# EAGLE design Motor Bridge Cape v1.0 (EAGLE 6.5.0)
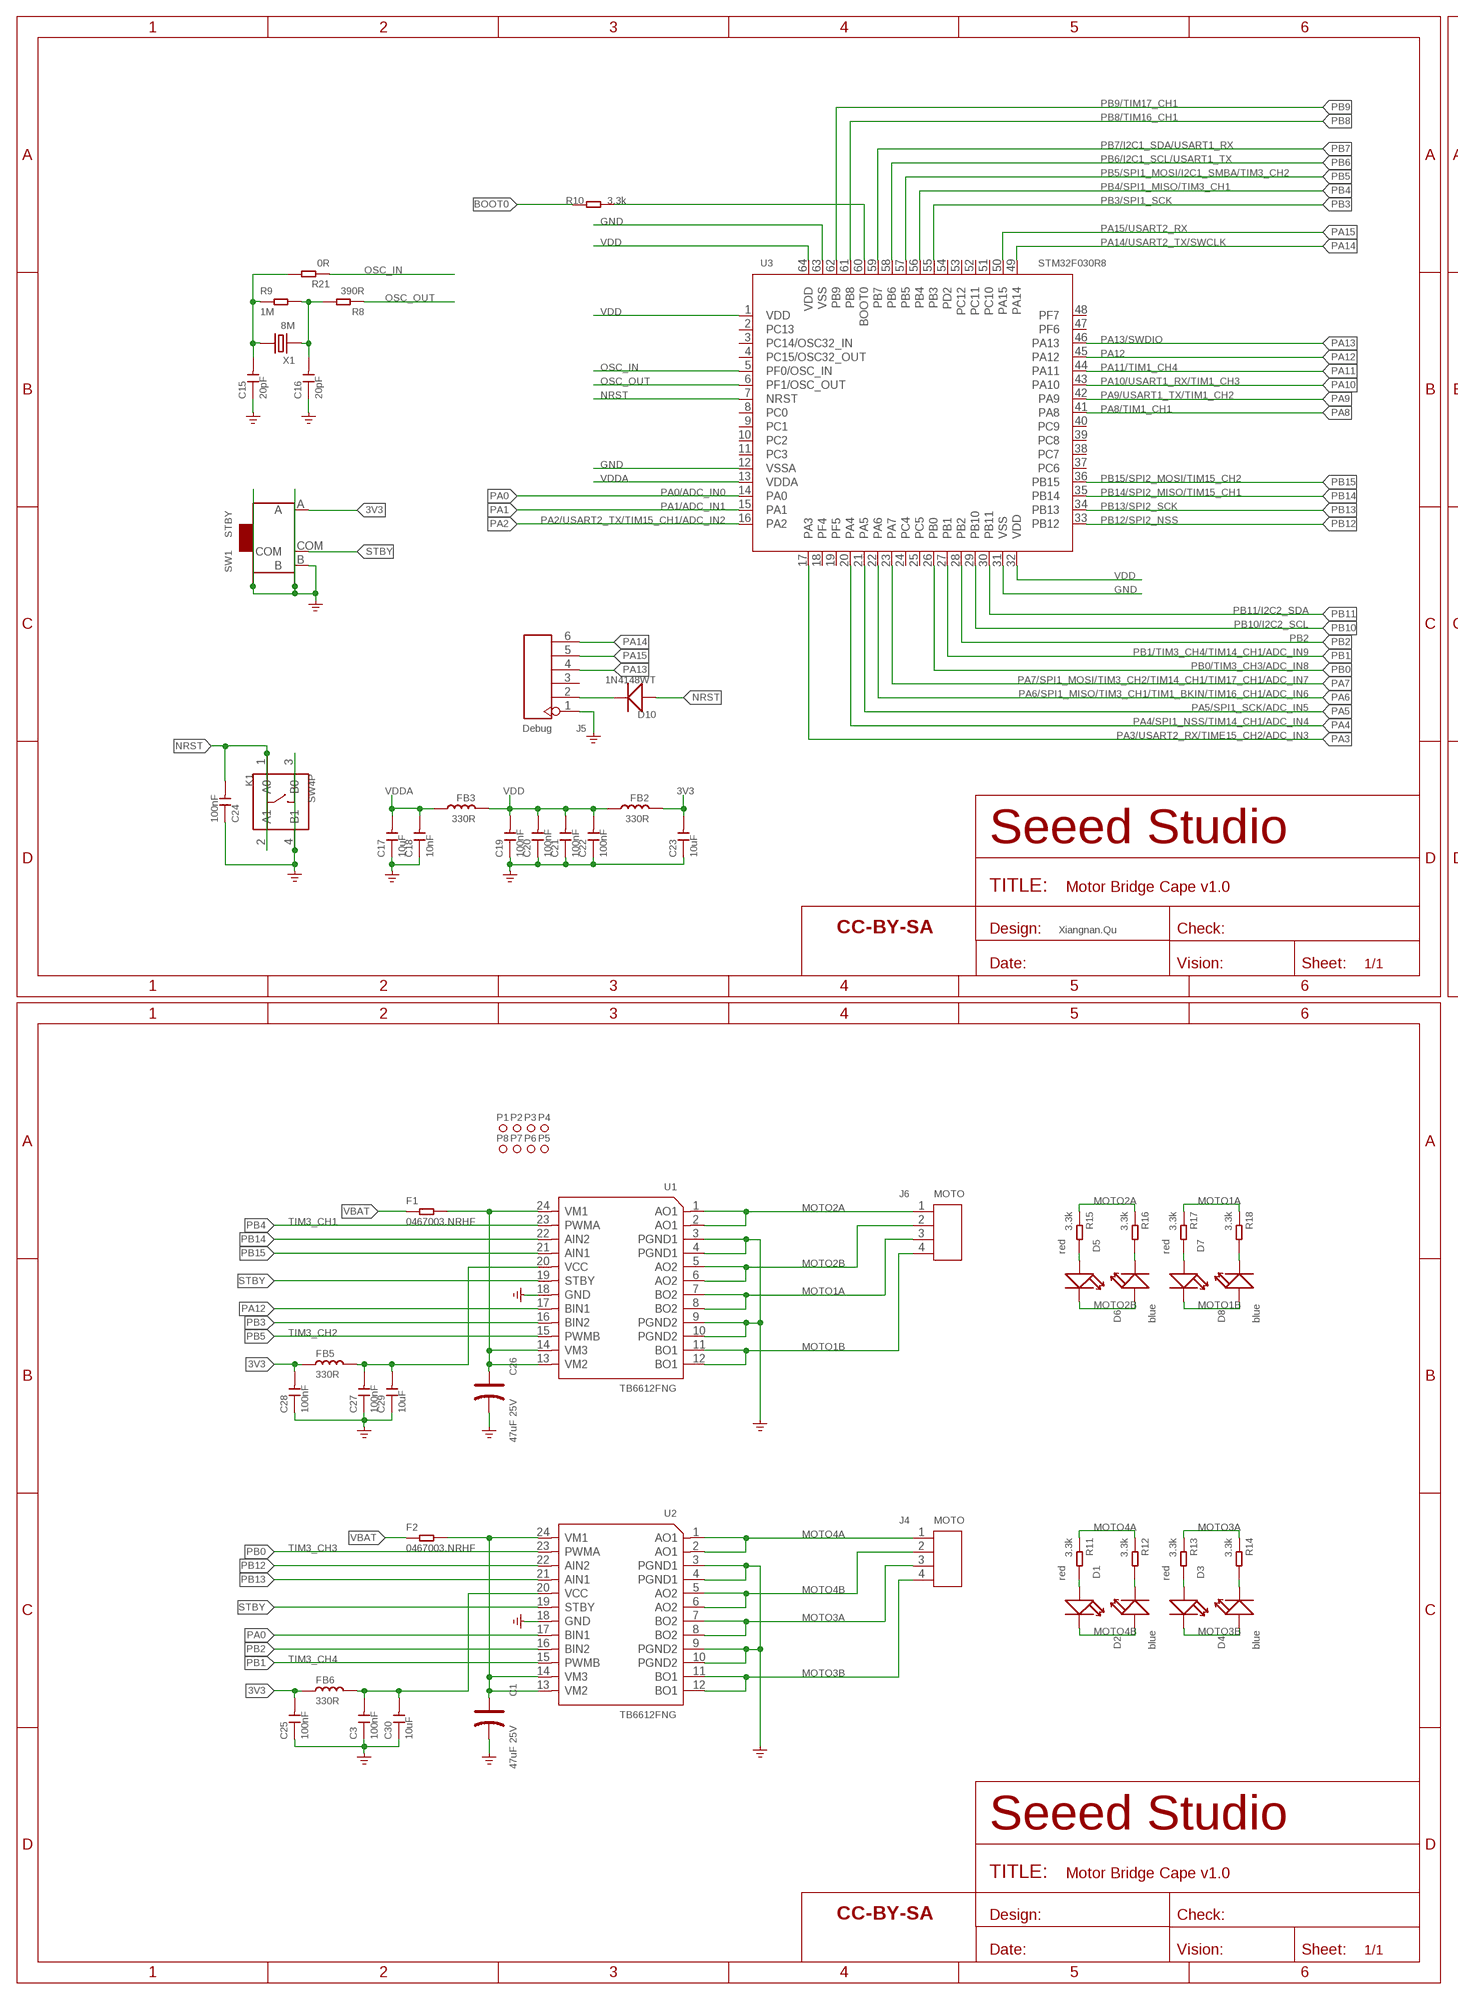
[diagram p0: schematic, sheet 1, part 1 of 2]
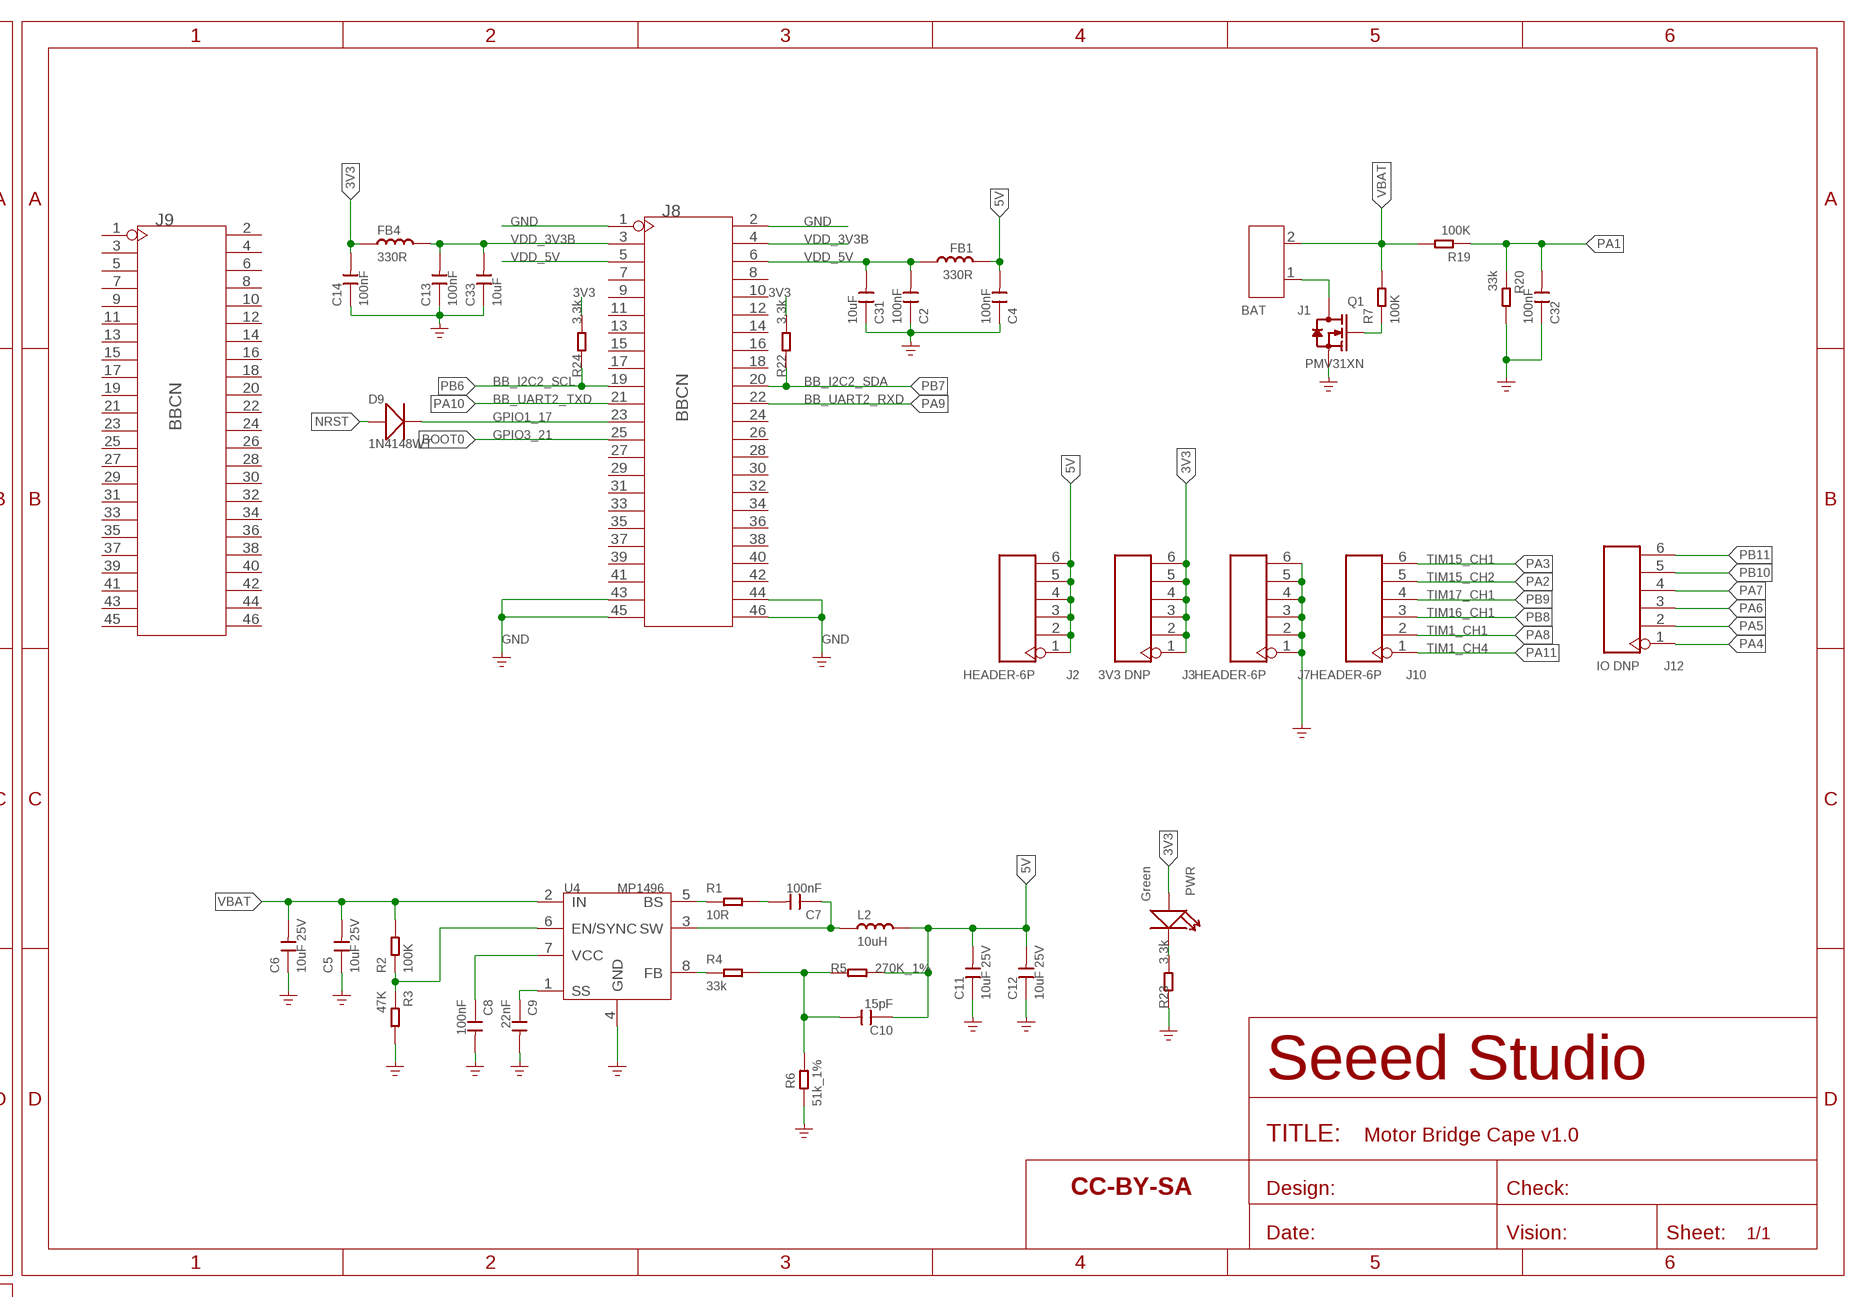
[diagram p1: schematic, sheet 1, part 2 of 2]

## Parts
C1  47uF 25V  CAP-POLAR-ELECTRO-C  [ELECTRO-SMD-C-6MM]
C2  100nF  CAP-0603  [C0603]
C3  100nF  CAP-0603  [C0603]
C4  100nF  CAP-0603  [C0603]
C5  10uF 25V  CAP-0805  [C0805]
C6  10uF 25V  CAP-0805  [C0805]
C7  100nF  CAP-0603  [C0603]
C8  100nF  CAP-0603  [C0603]
C9  22nF  CAP-0603  [C0603]
C10  15pF  CAP-0603  [C0603]
C11  10uF 25V  CAP-0805  [C0805]
C12  10uF 25V  CAP-0805  [C0805]
C13  100nF  CAP-0603  [C0603]
C14  100nF  CAP-0603  [C0603]
C15  20pF  CAP-0603  [C0603]
C16  20pF  CAP-0603  [C0603]
C17  10uF  CAP-0603  [C0603]
C18  10nF  CAP-0603  [C0603]
C19  100nF  CAP-0603  [C0603]
C20  100nF  CAP-0603  [C0603]
C21  100nF  CAP-0603  [C0603]
C22  100nF  CAP-0603  [C0603]
C23  10uF  CAP-0603  [C0603]
C24  100nF  CAP-0603  [C0603]
C25  100nF  CAP-0603  [C0603]
C26  47uF 25V  CAP-POLAR-ELECTRO-C  [ELECTRO-SMD-C-6MM]
C27  100nF  CAP-0603  [C0603]
C28  100nF  CAP-0603  [C0603]
C29  10uF  CAP-0603  [C0603]
C30  10uF  CAP-0603  [C0603]
C31  10uF  CAP-0603  [C0603]
C32  100nF  CAP-0603  [C0603]
C33  10uF  CAP-0603  [C0603]
D1  red  LED'0603'  [LED-0603]
D2  blue  LED'0603'  [LED-0603]
D3  red  LED'0603'  [LED-0603]
D4  blue  LED'0603'  [LED-0603]
D5  red  LED'0603'  [LED-0603]
D6  blue  LED'0603'  [LED-0603]
D7  red  LED'0603'  [LED-0603]
D8  blue  LED'0603'  [LED-0603]
D9  1N4148WT  DIODE'0603'  [SOD-523]
D10  1N4148WT  DIODE'0603'  [SOD-523]
F1  0467003.NRHF  RES-0603  [R0603]
F2  0467003.NRHF  RES-0603  [R0603]
FB1  330R  INDUCTOR/FERRITE-BEAD'0603'  [L0603]
FB2  330R  INDUCTOR/FERRITE-BEAD'0603'  [L0603]
FB3  330R  INDUCTOR/FERRITE-BEAD'0603'  [L0603]
FB4  330R  INDUCTOR/FERRITE-BEAD'0603'  [L0603]
FB5  330R  INDUCTOR/FERRITE-BEAD'0603'  [L0603]
FB6  330R  INDUCTOR/FERRITE-BEAD'0603'  [L0603]
FR1  SEEEDSTUDIO-OPEN-SCH-FRAME  [SEEEDSTUDIO-PCB-FRAME]
FR2  SEEEDSTUDIO-OPEN-SCH-FRAME  [SEEEDSTUDIO-PCB-FRAME]
FR4  SEEEDSTUDIO-OPEN-SCH-FRAME  [SEEEDSTUDIO-PCB-FRAME]
J1  BAT  SCREW-TERMINAL-2P'3.5'  [H2-3.5-7.0X7.0MM]
J2  HEADER-6P  HEADER-6P-65/35MIL  [H6-2.54-C65D35MIL]
J3  3V3 DNP  HEADER-6P-65/35MIL  [H6-2.54-C65D35MIL]
J4  MOTO  SCREW-TERMINAL-4P'3.5'  [H4-3.5-14.0X7.0MM]
J5  Debug  HEADER-6P-65/35MIL  [H6-2.54-C65D35MIL]
J6  MOTO  SCREW-TERMINAL-4P'3.5'  [H4-3.5-14.0X7.0MM]
J7  HEADER-6P  HEADER-6P-65/35MIL  [H6-2.54-C65D35MIL]
J8  BBCN  HEADER-2X23P  [2X23P-2.54]
J9  BBCN  HEADER-2X23P  [2X23P-2.54]
J10  HEADER-6P  HEADER-6P-65/35MIL  [H6-2.54-C65D35MIL]
J12  IO DNP  HEADER-6P-65/35MIL  [H6-2.54-C65D35MIL]
K1  SW4P  BUTTON-4P  [SW4P-SMD-4.5X3.2X2.5MM]
L2  10uH  INDUCTOR/FERRITE-BEAD'1813'  [L1813]
P1  MARK-1.0'ANNULAR'  [ROUND-MARK-1.0]
P2  MARK-1.0'ANNULAR'  [ROUND-MARK-1.0]
P3  MARK-1.0'ANNULAR'  [ROUND-MARK-1.0]
P4  MARK-1.0'ANNULAR'  [ROUND-MARK-1.0]
P5  MARK-1.0'ANNULAR'  [ROUND-MARK-1.0]
P6  MARK-1.0'ANNULAR'  [ROUND-MARK-1.0]
P7  MARK-1.0'ANNULAR'  [ROUND-MARK-1.0]
P8  MARK-1.0'ANNULAR'  [ROUND-MARK-1.0]
PWR  Green  LED'0603'  [LED-0603]
Q1  PMV31XN  MOSFET-N'SOT23'  [SOT-23]
R1  10R  RES-0603  [R0603]
R2  100K  RES-0603  [R0603]
R3  47K  RES-0603  [R0603]
R4  33k  RES-0603  [R0603]
R5  270K_1%  RES-0603  [R0603]
R6  51k_1%  RES-0603  [R0603]
R7  100K  RES-0603  [R0603]
R8  390R  RES-0603  [R0603]
R9  1M  RES-0603  [R0603]
R10  3.3k  RES-0603  [R0603]
R11  3.3k  RES-0603  [R0603]
R12  3.3k  RES-0603  [R0603]
R13  3.3k  RES-0603  [R0603]
R14  3.3k  RES-0603  [R0603]
R15  3.3k  RES-0603  [R0603]
R16  3.3k  RES-0603  [R0603]
R17  3.3k  RES-0603  [R0603]
R18  3.3k  RES-0603  [R0603]
R19  100K  RES-0603  [R0603]
R20  33k  RES-0603  [R0603]
R21  0R  RES-0603  [R0603]
R22  3.3k  RES-0603  [R0603]
R23  3.3k  RES-0603  [R0603]
R24  3.3k  RES-0603  [R0603]
SW1  STBY  SWITCH-3+4P  [SW7-SMD-L6.7X2.7X3.2MM]
U1  TB6612FNG  DRIVER-TB6612FNG  [SSOP24-0.65-8.3X5.6MM]
U2  TB6612FNG  DRIVER-TB6612FNG  [SSOP24-0.65-8.3X5.6MM]
U3  STM32F030R8  MCU-STM32F030R8  [LQFP64-0.5-10X10MM]
U4  MP1496  CONVERTER-MP1496DJ  [SOT-23-8]
X1  8M  CRYSTAL-2P'5032'  [X2-SMD-5.0X3.2X1.3MM]

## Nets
3V3: C14.2 C23.2 C25.2 C28.2 FB2.1 FB4.1 FB5.1 FB6.1 J3.1 J3.2 J3.3 J3.4 J3.5 J3.6 PWR.+ R22.1 R24.1 SW1.A
5V: C4.2 C10.1 C11.2 C12.2 FB1.1 J2.1 J2.2 J2.3 J2.4 J2.5 J2.6 L2.2 R5.2
BOOT0: J8.25 R10.2
GND: C1.- C2.1 C3.1 C4.1 C5.1 C6.1 C8.2 C9.2 C11.1 C12.1 C13.1 C14.1 C15.1 C16.1 C17.1 C18.1 C19.1 C20.1 C21.1 C22.1 C23.1 C24.1 C25.1 C26.- C27.1 C28.1 C29.1 C30.1 C31.1 C32.1 C33.1 J5.1 J7.1 J7.2 J7.3 J7.4 J7.5 J7.6 J8.1 J8.2 J8.43 J8.44 J8.45 J8.46 K1.3(B0) K1.4(B1) Q1.2(S) R3.2 R6.1 R20.2 R23.1 SW1.B SW1.SS1 SW1.SS2 SW1.SS3 SW1.SS4 U1.3(PGND1) U1.4(PGND1) U1.9(PGND2) U1.10(PGND2) U1.18(GND) U2.3(PGND1) U2.4(PGND1) U2.9(PGND2) U2.10(PGND2) U2.18(GND) U3.12(VSSA) U3.31(VSS) U3.63(VSS) U4.4(GND) ; supply symbol labelled GND_POWER
MOTO1A: J6.3 R17.1 R18.1 U1.7(BO2) U1.8(BO2)
MOTO1B: D7.- D8.+ J6.4 U1.11(BO1) U1.12(BO1)
MOTO2A: J6.1 R15.1 R16.1 U1.1(AO1) U1.2(AO1)
MOTO2B: D5.- D6.+ J6.2 U1.5(AO2) U1.6(AO2)
MOTO3A: J4.3 R13.1 R14.1 U2.7(BO2) U2.8(BO2)
MOTO3B: D3.- D4.+ J4.4 U2.11(BO1) U2.12(BO1)
MOTO4A: J4.1 R11.1 R12.1 U2.1(AO1) U2.2(AO1)
MOTO4B: D1.- D2.+ J4.2 U2.5(AO2) U2.6(AO2)
N$1: C10.2 R4.2 R5.1 R6.2
N$2: D3.+ R13.2
N$3: D4.- R14.2
N$4: C3.2 C30.2 FB6.2 U2.20(VCC)
N$5: R1.1 U4.5(BS)
N$6: C7.2 R1.2
N$7: C7.1 L2.1 U4.3(SW)
N$8: J1.1 Q1.3(D)
N$9: R4.1 U4.8(FB)
N$10: Q1.1(G) R7.1
N$11: D5.+ R15.2
N$12: C9.1 U4.1(SS)
N$13: C8.1 U4.7(VCC)
N$16: R2.1 R3.1 U4.6(EN/SYNC)
N$19: D1.+ R11.2
N$23: D2.- R12.2
N$24: D10.- J5.2
N$25: C16.2 R8.2 R9.2 X1.1
N$26: D6.- R16.2
N$27: C15.2 R9.1 R21.2 X1.2
N$28: R10.1 U3.60(BOOT0)
N$29: D7.+ R17.2
N$30: D8.- R18.2
N$31: C27.2 C29.2 FB5.2 U1.20(VCC)
N$32: C26.+ F1.2 U1.13(VM2) U1.14(VM3) U1.24(VM1)
N$34: C1.+ F2.2 U2.13(VM2) U2.14(VM3) U2.24(VM1)
N$44: PWR.- R23.2
N$60: D9.- J8.23
NRST: C24.2 D9.+ D10.+ K1.1(A0) K1.2(A1) U3.7(NRST)
OSC_IN: R21.1 U3.5(PF0/OSC_IN)
OSC_OUT: R8.1 U3.6(PF1/OSC_OUT)
PA0: U2.17(BIN1) U3.14(PA0)
PA1: C32.2 R19.1 R20.1 U3.15(PA1)
PA2: J10.5 U3.16(PA2)
PA3: J10.6 U3.17(PA3)
PA4: J12.1 U3.20(PA4)
PA5: J12.2 U3.21(PA5)
PA6: J12.3 U3.22(PA6)
PA7: J12.4 U3.23(PA7)
PA8: J10.2 U3.41(PA8)
PA9: J8.22 U3.42(PA9)
PA10: J8.21 U3.43(PA10)
PA11: J10.1 U3.44(PA11)
PA12: U1.17(BIN1) U3.45(PA12)
PA13: J5.4 U3.46(PA13)
PA14: J5.6 U3.49(PA14)
PA15: J5.5 U3.50(PA15)
PB0: U2.23(PWMA) U3.26(PB0)
PB1: U2.15(PWMB) U3.27(PB1)
PB2: U2.16(BIN2) U3.28(PB2)
PB3: U1.16(BIN2) U3.55(PB3)
PB4: U1.23(PWMA) U3.56(PB4)
PB5: U1.15(PWMB) U3.57(PB5)
PB6: J8.19 R24.2 U3.58(PB6)
PB7: J8.20 R22.2 U3.59(PB7)
PB8: J10.3 U3.61(PB8)
PB9: J10.4 U3.62(PB9)
PB10: J12.5 U3.29(PB10)
PB11: J12.6 U3.30(PB11)
PB12: U2.22(AIN2) U3.33(PB12)
PB13: U2.21(AIN1) U3.34(PB13)
PB14: U1.22(AIN2) U3.35(PB14)
PB15: U1.21(AIN1) U3.36(PB15)
STBY: SW1.COM U1.19(STBY) U2.19(STBY)
VBAT: C5.2 C6.2 F1.1 F2.1 J1.2 R2.2 R7.2 R19.2 U4.2(IN)
VDD: C19.2 C20.2 C21.2 C22.2 FB2.2 FB3.1 U3.1(VDD) U3.32(VDD) U3.64(VDD)
VDD_3V3B: C13.2 C33.2 FB4.2 J8.3 J8.4
VDD_5V: C2.2 C31.2 FB1.2 J8.5 J8.6
VDDA: C17.2 C18.2 FB3.2 U3.13(VDDA)
Unconnected: J5.3 J8.7 J8.8 J8.9 J8.10 J8.11 J8.12 J8.13 J8.14 J8.15 J8.16 J8.17 J8.18 J8.24 J8.26 J8.27 J8.28 J8.29 J8.30 J8.31 J8.32 J8.33 J8.34 J8.35 J8.36 J8.37 J8.38 J8.39 J8.40 J8.41 J8.42 J9.1 J9.2 J9.3 J9.4 J9.5 J9.6 J9.7 J9.8 J9.9 J9.10 J9.11 J9.12 J9.13 J9.14 J9.15 J9.16 J9.17 J9.18 J9.19 J9.20 J9.21 J9.22 J9.23 J9.24 J9.25 J9.26 J9.27 J9.28 J9.29 J9.30 J9.31 J9.32 J9.33 J9.34 J9.35 J9.36 J9.37 J9.38 J9.39 J9.40 J9.41 J9.42 J9.43 J9.44 J9.45 J9.46 U3.2(PC13) U3.3(PC14/OSC32_IN) U3.4(PC15/OSC32_OUT) U3.8(PC0) U3.9(PC1) U3.10(PC2) U3.11(PC3) U3.18(PF4) U3.19(PF5) U3.24(PC4) U3.25(PC5) U3.37(PC6) U3.38(PC7) U3.39(PC8) U3.40(PC9) U3.47(PF6) U3.48(PF7) U3.51(PC10) U3.52(PC11) U3.53(PC12) U3.54(PD2)

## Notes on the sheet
- PB9/TIM17_CH1
- PB8/TIM16_CH1
- PB7/I2C1_SDA/USART1_RX
- PB6/I2C1_SCL/USART1_TX
- PB5/SPI1_MOSI/I2C1_SMBA/TIM3_CH2
- PB4/SPI1_MISO/TIM3_CH1
- PB3/SPI1_SCK
- PA15/USART2_RX
- PA14/USART2_TX/SWCLK
- BB_I2C2_SCL | BB_I2C2_SDA
- BB_UART2_TXD | BB_UART2_RXD
- GPIO1_17
- PA13/SWDIO | GPIO3_21
- PA12
- PA11/TIM1_CH4
- PA10/USART1_RX/TIM1_CH3
- PA9/USART1_TX/TIM1_CH2
- PA8/TIM1_CH1
- TIM15_CH1
- TIM15_CH2
- TIM17_CH1
- PB15/SPI2_MOSI/TIM15_CH2 | TIM16_CH1
- PA0/ADC_IN0 | PB14/SPI2_MISO/TIM15_CH1 | TIM1_CH1
- PA1/ADC_IN1 | PB13/SPI2_SCK | TIM1_CH4
- PA2/USART2_TX/TIM15_CH1/ADC_IN2 | PB12/SPI2_NSS
- PB11/I2C2_SDA
- PB10/I2C2_SCL
- PB2
- PB1/TIM3_CH4/TIM14_CH1/ADC_IN9
- PB0/TIM3_CH3/ADC_IN8
- PA7/SPI1_MOSI/TIM3_CH2/TIM14_CH1/TIM17_CH1/ADC_IN7
- PA6/SPI1_MISO/TIM3_CH1/TIM1_BKIN/TIM16_CH1/ADC_IN6
- PA5/SPI1_SCK/ADC_IN5
- PA4/SPI1_NSS/TIM14_CH1/ADC_IN4
- PA3/USART2_RX/TIME15_CH2/ADC_IN3
- Xiangnan.Qu
- TIM3_CH1
- TIM3_CH2
- TIM3_CH3
- TIM3_CH4

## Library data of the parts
C1 C26 = Discrete-new:CAP-POLAR: Electrolytic Capacitors,Tantalum Capacitors and Super Capacitors
C2-C25 C27-C33 = Discrete-new:CAP: Ceramic Capacitors
D1-D8 PWR = Discrete-new:LED
D9 D10 = Discrete-new:DIODE*
F1 F2 R1-R24 = Discrete-new:RES
FB1-FB6 L2 = Discrete-new:INDUCTOR/FERRITE-BEAD
FR1 FR2 FR4 = moudle-new:SEEEDSTUDIO-OPEN-SCH-FRAME
J1 = Connector-new:SCREW-TERMINAL-2P: 2P-3.5:320110028;2P-5.0:320110031
J2 J3 J5 J7 J10 J12 = Connector-new:HEADER-6P
J4 J6 = Connector-new:SCREW-TERMINAL-4P: 203000033
J8 J9 = Connector :HEADER-2X23P
K1 = Discrete-new:BUTTON-4P: SW4-6.0X6.0X5.0MM:311020024;SW4-8.0X8.0X9.0MM:311020028;SW4-SMD-6.0X6.0X5.0MM:311020004;SW4-SMD-3.35X3.35X1.5MM:311020030;SW4-SMD-5.2X5.2X2.5MM:311020046
P1-P8 = Discrete-new:MARK-1.0; PARTNO: DNP
Q1 = Discrete-new:MOSFET-N
SW1 = Discrete-new:SWITCH-3+4P: SW7-SMD-6.7X2.6X1.4MM-90D:311030002;SW7-SMD-L6.7X2.7X3.2MM:311030001
U1 U2 = template:DRIVER-TB6612FNG; MPN: TB6612FNG
U3 = IC-new:MCU-STM32F030R8
U4 = template:CONVERTER-MP1496DJ: High-Efficiency,2A，16V,500kHz Synchronous,Step-Down Converter http://html.alldatasheetcn.com/html-pdf/551584/MPS/MP1496DJ/55/1/MP1496DJ.html
X1 = Discrete-new:CRYSTAL-2P

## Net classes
0 default: width 0.152 mm, drill 0.305 mm, clearance 0.152 mm

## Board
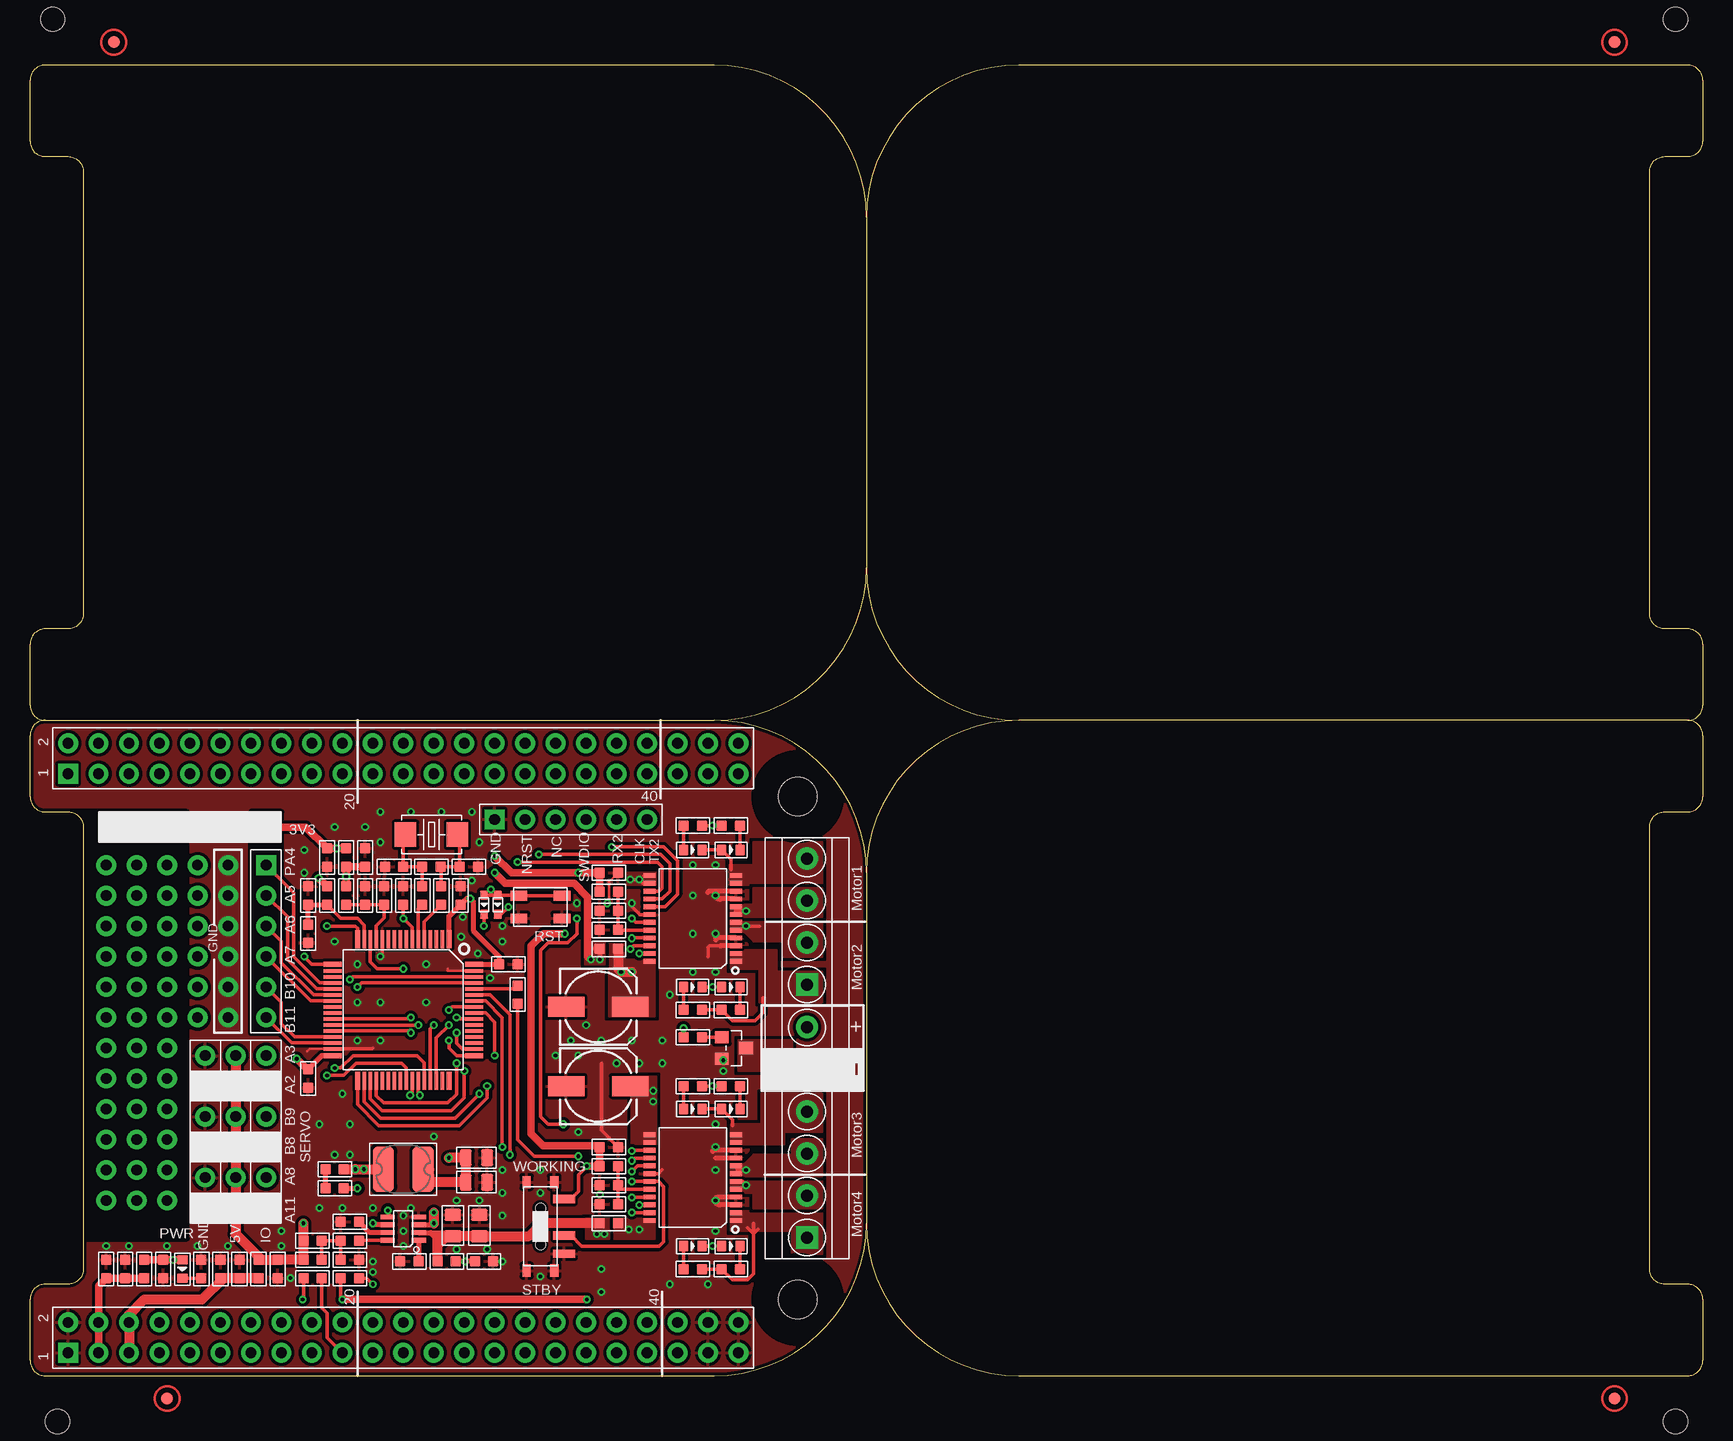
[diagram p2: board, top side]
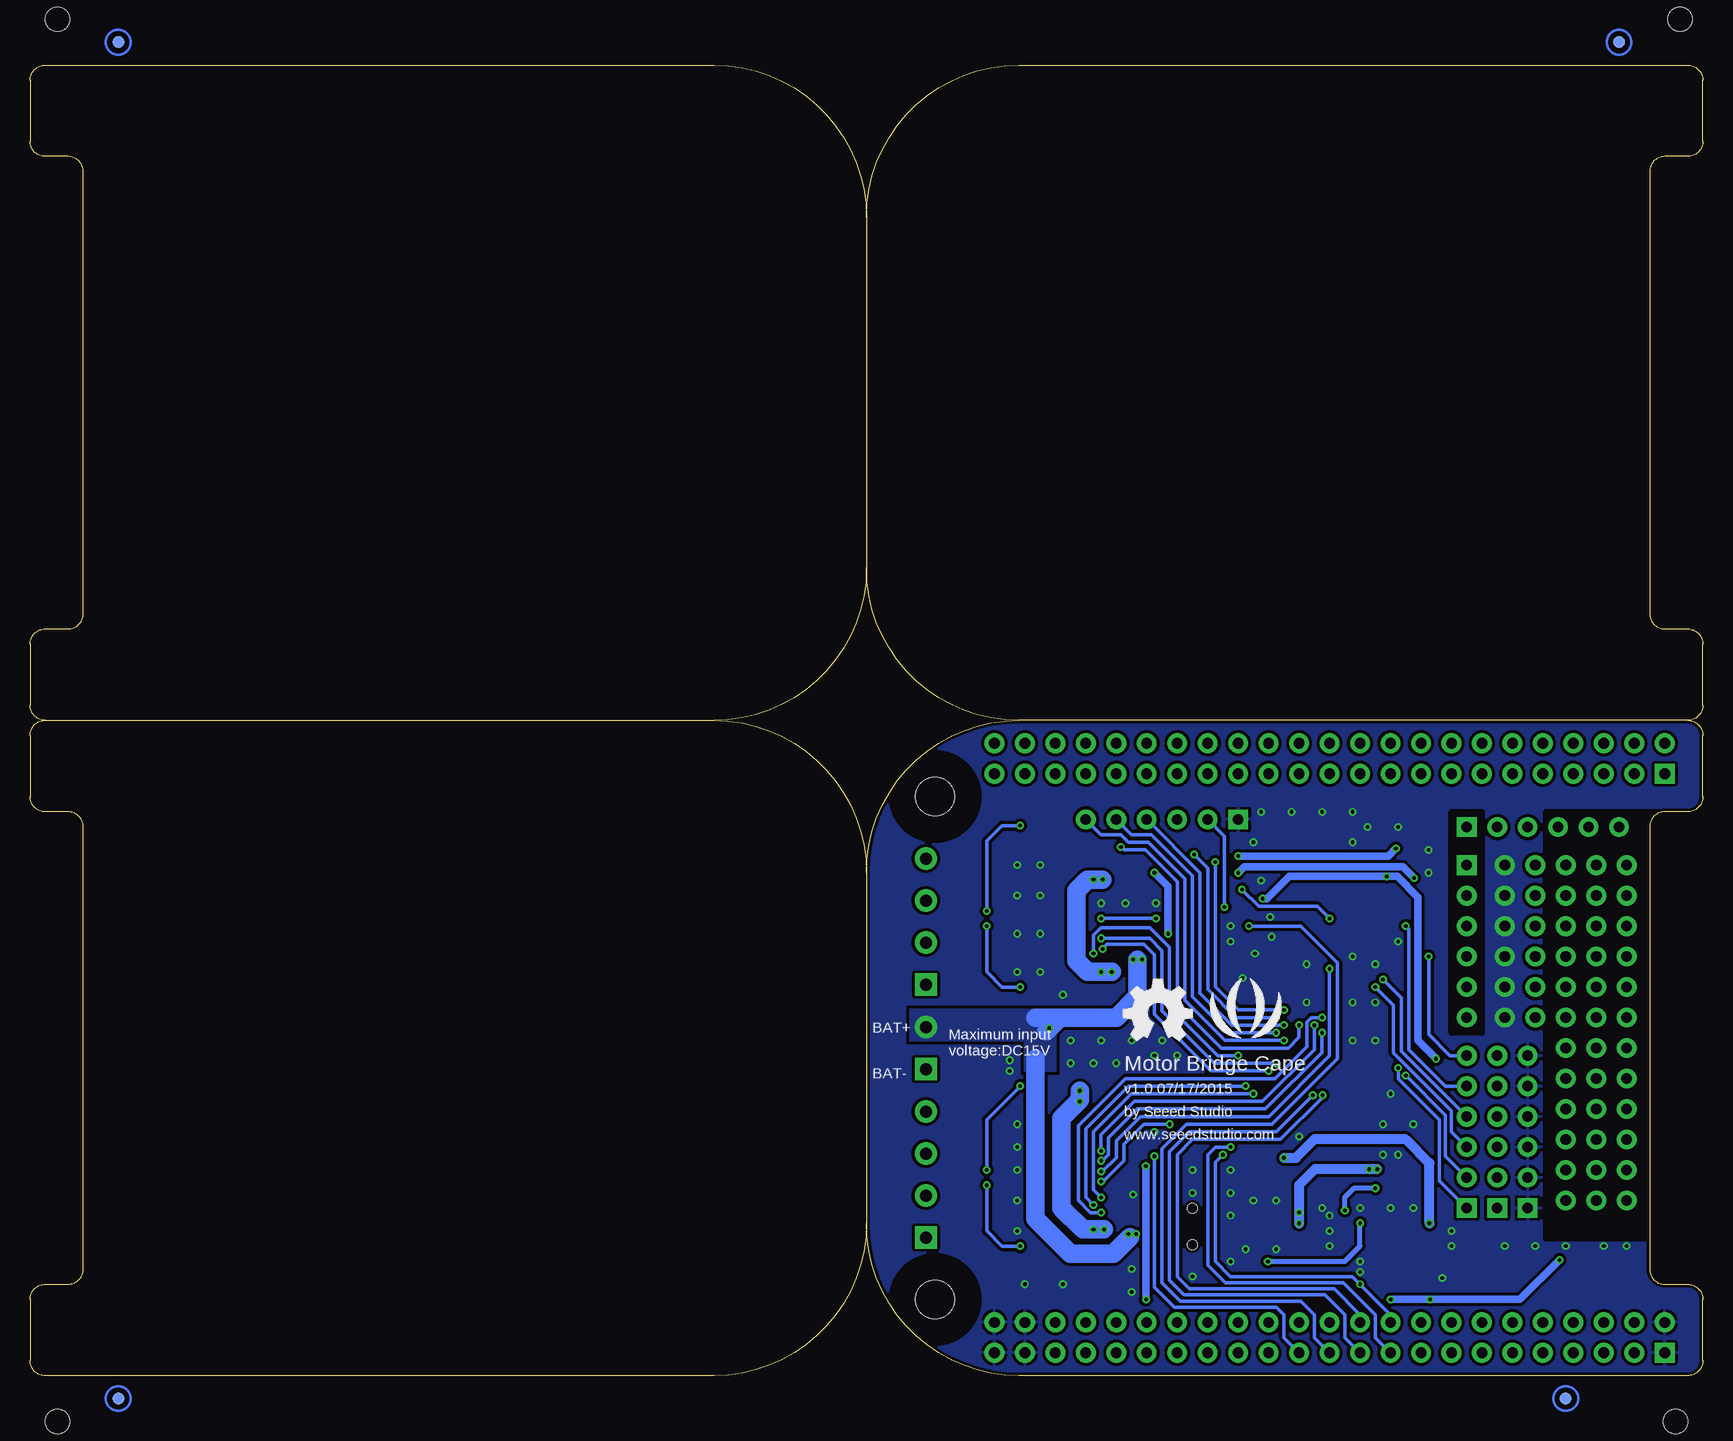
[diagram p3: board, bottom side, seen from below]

Size 139.45 x 109.22 mm. Coordinates in mm from the lower left corner, seen from the top.
Outline: 64 segments
Copper layers (1*16): Top 0.035mm / dielectric 1.5mm / Bottom 0.035mm
Design rules "SeeedStudio_2layer_DRU_no_angle_20140221 *": minimum track width 6mil, minimum drill 12mil, track to track 6mil, track to pad 6mil, pad to pad 6mil, via to via 6mil, smd to smd 0mil, copper to edge 10mil, drill to drill 10mil, minimum pad ring 10mil, minimum via ring 6mil, stop-mask expansion 2mil, vias tented up to drill 25mil, thermal gap 10mil
Holes 2 mm at 1.91,113.03 137.16,113.03 2.29,-3.81 137.16,-3.81
tRestrict: area 18.4,28.6 to 21,47; area 2.5,11.4 to 13.1,47
bRestrict: area 18.4,28.6 to 21,47; area 2.5,11.4 to 13.1,47

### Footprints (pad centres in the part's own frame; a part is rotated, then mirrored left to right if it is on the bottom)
ELECTRO-SMD-C-6MM = smd 3.048 x 1.651: + 2.667,0; - -2.667,0
C0603 = smd 0.889 x 0.889: 1 0,0.762; 2 0,-0.762
C0805 = smd 1.397 x 1.016: 1 0,0.889; 2 0,-0.889
LED-0603 = smd 0.762 x 0.889: + -0.762,0; - 0.762,0
SOD-523 = smd 0.762 x 0.7: + -0.8,0; - 0.8,0
R0603 = smd 0.889 x 0.889: 1 0,0.762; 2 0,-0.762
L0603 = smd 0.889 x 0.889: 1 -0.762,0; 2 0.762,0
H2-3.5-7.0X7.0MM = drill 1 pad 1.85 square: 1 -1.75,0 | drill 1 pad 1.85: 2 1.75,0
H6-2.54-C65D35MIL = drill 0.889 pad 1.651 square: 1 0,6.35 | drill 0.889 pad 1.651: 2 0,3.81; 3 0,1.27; 4 0,-1.27; 5 0,-3.81; 6 0,-6.35
H4-3.5-14.0X7.0MM = drill 1 pad 1.85 square: 1 -5.25,0 | drill 1 pad 1.85: 2 -1.75,0; 3 1.75,0; 4 5.25,0
2X23P-2.54 = drill 0.889 pad 1.651 square: 1 -1.27,27.94 | drill 0.889 pad 1.651: 2 1.27,27.94; 3 -1.27,25.4; 4 1.27,25.4; 5 -1.27,22.86; 6 1.27,22.86; 7 -1.27,20.32; 8 1.27,20.32; 9 -1.27,17.78; 10 1.27,17.78; 11 -1.27,15.24; 12 1.27,15.24; 13 -1.27,12.7; 14 1.27,12.7; 15 -1.27,10.16; 16 1.27,10.16; 17 -1.27,7.62; 18 1.27,7.62; 19 -1.27,5.08; 20 1.27,5.08; 21 -1.27,2.54; 22 1.27,2.54; 23 -1.27,0; 24 1.27,0; 25 -1.27,-2.54; 26 1.27,-2.54; 27 -1.27,-5.08; 28 1.27,-5.08; 29 -1.27,-7.62; 30 1.27,-7.62; 31 -1.27,-10.16; 32 1.27,-10.16; 33 -1.27,-12.7; 34 1.27,-12.7; 35 -1.27,-15.24; 36 1.27,-15.24; 37 -1.27,-17.78; 38 1.27,-17.78; 39 -1.27,-20.32; 40 1.27,-20.32; 41 -1.27,-22.86; 42 1.27,-22.86; 43 -1.27,-25.4; 44 1.27,-25.4; 45 -1.27,-27.94; 46 1.27,-27.94
SW4P-SMD-4.5X3.2X2.5MM = smd 1.4 x 0.8: 1 -1.8,-0.94; 2 1.8,-0.94; 3 1.8,0.94; 4 -1.8,0.94
L1813 = smd 1.778 x 3.81: 1 -1.651,0; 2 1.651,0
ROUND-MARK-1.0 = smd 1.016 x 1.016: P$1 0,0
SOT-23 = smd 1.016 x 1.143: 1 -0.889,-1.016; 2 0.889,-1.016; 3 0,1.016
SW7-SMD-L6.7X2.7X3.2MM = smd 1.8 x 0.7: A 1.978,2.286; B 1.978,-2.286; COM 1.978,-0.762 | smd 0.7 x 1.016: SS1 -1.15,-3.683; SS2 1.15,-3.683; SS3 1.15,3.683; SS4 -1.15,3.683 | hole 0.813: 0,-1.524; 0,1.524
SSOP24-0.65-8.3X5.6MM = smd 0.4 x 1: 1 -3.575,-3.6; 2 -2.925,-3.6; 3 -2.275,-3.6; 4 -1.625,-3.6; 5 -0.975,-3.6; 6 -0.325,-3.6; 7 0.325,-3.6; 8 0.975,-3.6; 9 1.625,-3.6; 10 2.275,-3.6; 11 2.925,-3.6; 12 3.575,-3.6; 13 3.575,3.6; 14 2.925,3.6; 15 2.275,3.6; 16 1.625,3.6; 17 0.975,3.6; 18 0.325,3.6; 19 -0.325,3.6; 20 -0.975,3.6; 21 -1.625,3.6; 22 -2.275,3.6; 23 -2.925,3.6; 24 -3.575,3.6
LQFP64-0.5-10X10MM = smd 1.5 x 0.4: 1 -5.9,3.81; 16 -5.9,-3.81; 33 5.9,-3.81; 48 5.9,3.81 | smd 1.5 x 0.28: 2 -5.9,3.25; 3 -5.9,2.75; 4 -5.9,2.25; 5 -5.9,1.75; 6 -5.9,1.25; 7 -5.9,0.75; 8 -5.9,0.25; 9 -5.9,-0.25; 10 -5.9,-0.75; 11 -5.9,-1.25; 12 -5.9,-1.75; 13 -5.9,-2.25; 14 -5.9,-2.75; 15 -5.9,-3.25; 34 5.9,-3.25; 35 5.9,-2.75; 36 5.9,-2.25; 37 5.9,-1.75; 38 5.9,-1.25; 39 5.9,-0.75; 40 5.9,-0.25; 41 5.9,0.25; 42 5.9,0.75; 43 5.9,1.25; 44 5.9,1.75; 45 5.9,2.25; 46 5.9,2.75; 47 5.9,3.25 | smd 0.4 x 1.5: 17 -3.81,-5.9; 32 3.81,-5.9; 49 3.81,5.9; 64 -3.81,5.9 | smd 0.28 x 1.5: 18 -3.25,-5.9; 19 -2.75,-5.9; 20 -2.25,-5.9; 21 -1.75,-5.9; 22 -1.25,-5.9; 23 -0.75,-5.9; 24 -0.25,-5.9; 25 0.25,-5.9; 26 0.75,-5.9; 27 1.25,-5.9; 28 1.75,-5.9; 29 2.25,-5.9; 30 2.75,-5.9; 31 3.25,-5.9; 50 3.25,5.9; 51 2.75,5.9; 52 2.25,5.9; 53 1.75,5.9; 54 1.25,5.9; 55 0.75,5.9; 56 0.25,5.9; 57 -0.25,5.9; 58 -0.75,5.9; 59 -1.25,5.9; 60 -1.75,5.9; 61 -2.25,5.9; 62 -2.75,5.9; 63 -3.25,5.9
SOT-23-8 = smd 0.4 x 1.2: 1 -0.975,-1.3; 2 -0.325,-1.3; 3 0.325,-1.3; 4 0.975,-1.3; 5 0.975,1.3; 6 0.325,1.3; 7 -0.325,1.3; 8 -0.975,1.3
HOLE-3.2/7.0 = hole 3.2: 0,0
X2-SMD-5.0X3.2X1.3MM = smd 1.778 x 2.032: 1 -2.159,0; 2 2.159,0

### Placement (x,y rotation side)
C1  47.37,24.13 0 top
C2  15.88,8.89 0 top
C3  48.26,14.29 90 top
C4  20.64,8.89 180 top
C5  35.24,12.51 0 top
C6  37.47,12.51 0 top
C7  25.4,17.21 270 top
C8  26.67,12.83 270 top
C9  31.62,9.53 270 top
C10  23.56,9.65 90 top
C11  37.21,16.13 270 top
C12  37.21,18.16 270 top
C13  6.35,8.89 0 top
C14  11.11,8.89 180 top
C15  36.58,42.42 270 top
C16  30.35,42.42 90 top
C17  29.53,40.01 0 top
C18  27.94,40.01 0 top
C19  23.18,24.77 180 top
C20  27.94,43.18 0 top
C21  39.88,34.29 270 top
C22  35.88,40.01 0 top
C23  24.77,43.18 180 top
C24  31.11,40.01 0 top
C25  48.26,19.05 270 top
C26  47.37,30.73 0 top
C27  48.26,37.15 90 top
C28  48.26,41.91 270 top
C29  48.26,38.73 90 top
C30  48.26,15.88 90 top
C31  17.46,8.89 0 top
C32  23.18,40.01 0 top
C33  7.94,8.89 0 top
D1  55.24,10.79 0 top
D2  58.42,10.79 0 top
D3  55.24,22.23 0 top
D4  58.42,22.23 0 top
D5  55.24,32.38 0 top
D6  58.42,32.38 0 top
D7  55.24,43.81 0 top
D8  58.42,43.81 0 top
D9  37.85,39.24 270 top
D10  38.99,39.24 270 top
F1  48.26,35.56 90 top
F2  48.26,12.7 90 top
FB1  19.05,8.89 270 top
FB2  26.35,43.18 270 top
FB3  26.35,40.01 270 top
FB4  9.53,8.89 270 top
FB5  48.26,40.32 0 top
FB6  48.26,17.46 0 top
FR1  not placed on the board
FR2  not placed on the board
FR4  not placed on the board
J1  64.77,27.3 90 top
J2  17.14,20.32 180 top
J3  13.34,45.72 270 top
J4  64.77,16.76 90 top
J5  45.09,46.35 90 top
J6  64.77,37.85 90 top
J7  14.61,20.32 180 top
J8  31.11,3.17 90 top
J9  31.11,51.44 90 top
J10  19.68,20.32 180 top
J12  19.68,36.2 0 top
K1  42.55,39.05 180 top
L2  31.11,17.21 0 top
P1  11.43,-1.91 0 top
P2  11.43,-1.91 0 bottom
P3  132.08,-1.91 0 top
P4  132.08,-1.91 0 bottom
P5  6.99,111.12 90 top
P6  6.99,111.12 270 bottom
P7  132.08,111.12 90 top
P8  132.08,111.12 270 bottom
PWR  12.7,8.89 270 top
Q1  58.67,27.3 270 top
R1  25.4,15.62 270 top
R2  34.73,9.53 270 top
R3  37.85,9.53 90 top
R4  26.67,11.24 270 top
R5  23.56,11.24 270 top
R6  26.67,9.65 270 top
R7  55.24,28.19 270 top
R8  32.7,40.01 180 top
R9  33.46,42.42 270 top
R10  40.64,31.75 0 top
R11  55.24,8.89 270 top
R12  58.42,8.89 90 top
R13  55.24,24.13 270 top
R14  58.42,24.13 90 top
R15  55.24,30.48 270 top
R16  58.42,30.48 90 top
R17  55.24,45.85 270 top
R18  58.42,45.85 90 top
R19  24.77,40.01 180 top
R20  23.18,36.83 0 top
R21  34.29,40.01 180 top
R22  26.67,8.13 90 top
R23  14.29,8.89 0 top
R24  23.56,8.13 90 top
SW1  42.55,12.45 0 top
U1  55.24,38.1 90 top
U2  55.24,16.51 90 top
U3  31.11,30.48 270 top
U4  31.11,12.26 90 top
U$16  [SEEED-SILK-280*268MIL]  38.1,29.84 0 bottom
U$18  [OSHW_FILLX200_NOTEXT]  48.26,27.94 0 bottom
U$26  [HOLE-3.2/7.0]  64.01,48.26 0 top
U$27  [HOLE-3.2/7.0]  64.01,6.35 0 top
X1  33.46,45.09 0 top

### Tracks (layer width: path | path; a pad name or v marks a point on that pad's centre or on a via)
3V3  (via drill 0.3, 0.3 pad 0.64)
  Top 0.305: SW1.A 45.09,14.73 45.72,15.37 45.72,16.75 v46.43,17.46 | R24.1 22.8,6.41 v22.73,6.35 | R22.1 25.91,6.48 v26.04,6.35
  Top 0.61: J3.6 J3.5 J3.4 J3.3 J3.2 J3.1 22.99,45.72 C23.2 v25.59,43.94 FB2.1 | PWR.+ v11.94,9.65 C14.2 FB4.1 | FB5.1 C28.2 v45.72,41.91 40.13,41.91 v38.73,43.31 | v46.43,17.46 FB6.1 47.5,18.8 47.37,18.92 C25.2 47.5,19.18 42.77,19.18 41.78,20.17 41.78,35.81 42.8,36.83 v44.58,36.83 | v46.42,6.35 v26.04,6.35
  Bottom 0.61: v38.73,43.31 26.23,43.31 v25.59,43.94 | v44.58,36.83 44.58,40.77 v45.72,41.91 | v46.42,6.35 46.42,17.45 v46.43,17.46 | v26.04,6.35 v22.73,6.35 15.24,6.35 v11.94,9.65
5V  (via drill 0.3 pad 0.64)
  Top 0.813: J2.6 J2.5 | 17.14,24 J2.5 | J2.5 J2.4 J2.3 J2.2 J2.1 17.14,11.81 19.3,9.65 | FB1.1 19.3,9.65 | 19.3,9.65 C4.2 C10.1 R5.2 v22.8,12.7 | v34.92,18.16 C12.2 C11.2 33.27,16.13 33.27,16.26 33.27,16.7 | 33.27,16.7 33.27,17.19 | L2.2 33.27,16.7
  Bottom 0.813: v22.8,12.7 22.8,17.72 24.77,19.68 32.38,19.68 33.91,18.16 v34.92,18.16
BOOT0  (via drill 0.3 pad 0.64)
  Top 0.305: R10.2 40.64,19.67 42.02,18.29 v45.72,18.29
  Bottom 0.305: J8.25 34.92,3.17 34.92,5.08 35.56,5.71 44.07,5.71 45.72,7.37 v45.72,18.29
GND  (via drill 0.3 pad 0.64, 0.89 pad 1.65)
  Top 0.203: C28.1 48.26,41.15 48.26,39.5 48.2,39.43 | v48.13,39.37 C29.1 47.37,38.61 | U3.31 23.29,27.23 23.11,27.05 | U3.63 34.8,33.73 34.8,33.91
  Top 0.305: U2.18 52.4,16.84 52.7,17.14 | C25.1 47.62,20.45 47.62,26.04 | U3.31 28.5,27.23 28.57,27.3 | U3.12 29.36,35.08 v29.21,34.92 | U1.3 56.65,35.83 56.52,35.69 56.52,34.92 | U1.4 57.25,36.48 57.15,36.58 | U1.9 58.72,39.73 57.63,39.73 57.53,39.62 | U1.18 50.86,38.42 50.16,39.12 | v48.13,39.37 48.2,39.43 | U2.4 58.82,14.86 57.15,14.86
  Top 0.406: U2.4 57.43,14.88 arc90 v57.15,14.61 arc90 57.52,14.23 U2.3 | U2.9 57.18,18.14 arc-90 57.15,18.16 | U2.10 57.01,18.79 arc90 56.9,18.67 | U1.3 57.54,35.83 arc90 57.53,35.81 | U1.4 57.3,36.48 arc90 57.15,36.32 | U1.10 56.63,40.38 arc90 56.52,40.26 | 58.72,39.73 57.43,39.73 arc-90 57.28,39.88
  other vias: 31.11,13.34 31.11,12.06 31.11,10.79 28.57,9.53 26.04,13.97 28.57,13.97 24.13,13.97 31.75,13.97 35.56,14.61 37.47,14.61 39.37,15.24 39.37,13.34 39.37,17.14 35.56,10.54 39.37,9.53 27.3,27.94 29.21,27.94 27.3,31.11 29.21,31.11 25.4,36.2 27.3,34.29 22.86,41.91 22.86,43.81 33.02,31.11 33.02,34.29 36.83,41.27 37.47,44.45 29.21,44.45 25.4,45.72 27.94,45.72 29.21,46.99 31.75,46.99 34.29,46.99 36.83,46.99 45.59,39.37 50.16,39.37 43.81,26.67 45.72,26.67 50.8,26.04 47.62,27.94 50.16,27.94 45.09,27.94 45.72,20.32 47.5,15.11 55.24,40.01 55.24,42.55 42.55,8.26 42.55,17.14 42.55,15.24 47.62,8.89 47.62,6.99 56.52,7.62 53.34,7.62 6.35,10.79 8.26,10.79 13.97,10.79 16.51,10.79 11.43,10.79 20.95,10.79 24.13,20.95 26.67,20.95 26.67,18.41 33.66,19.94 25.4,18.41 38.1,10.54 57.15,19.05 57.15,40.01 57.15,42.55 57.15,36.83 55.24,36.83 55.24,33.66 57.15,33.66 57.15,20.95 57.15,17.14 57.15,12.06 52.7,27.94 57.78,26.29 57.78,25.4 46.35,29.21 52.7,26.04 53.34,31.75 26.04,23.5 48.9,26.04 16.51,42.55 16.51,40.01 16.51,37.47 16.51,34.92 16.51,32.38 16.51,29.84 38.35,33.15 28.57,8.64 21.72,8.13 20.95,12.06 39.37,37.47 39.37,36.2 37.34,35.18 35.94,36.58 36.07,38.23
  pour Top (isolate 0.254, rank 6): 0,54.61 69.85,54.61 69.85,0 0,0
  pour Bottom (isolate 0.254, rank 6): 0,54.61 69.85,54.61 69.85,0 0,0
  pour Top (isolate 0.254, no thermals): 58.42,25.4 58.42,27.3 56.52,27.3 56.52,25.4
MOTO1A  (via drill 0.3 pad 0.64)
  Top 0.305: R18.1 v56.9,45.85 R17.1 | v59.69,38.73 58.8,38.73 58.8,38.47 U1.7
  Bottom 0.305: v59.69,38.73 59.69,44.58 58.42,45.85 v56.9,45.85
  pour Top (isolate 0.254, no thermals): 58.42,38.23 66.04,38.23 66.04,40.64 60.33,40.64 60.33,39.24 58.42,39.24
MOTO1B
  Top 0.305: D7.- D8.+ 58.42,43.05 58.42,42.16
  pour Top (isolate 0.254, rank 2, no thermals): 58.29,40.89 58.29,42.55 60.33,42.55 60.33,44.45 66.04,44.45 66.04,40.89
MOTO2A
  Top 0.305: R15.1 R16.1 58.55,29.59 60.45,29.59 61.09,30.23 61.09,31.5
  pour Top (isolate 0.254, no thermals): 58.42,35.43 62.23,35.43 62.23,33.66 66.04,33.66 66.04,31.11 60.83,31.11 60.83,33.91 58.42,33.91
MOTO2B  (via drill 0.3 pad 0.64)
  Top 0.305: D6.+ v56.9,32.38 D5.- | v59.69,37.47 60.83,37.47
  Bottom 0.305: v56.9,32.38 58.42,32.38 59.69,33.66 v59.69,37.47
  pour Top (isolate 0.254, rank 2, no thermals): 58.42,37.97 58.42,36.96 59.56,36.96 60.33,36.2 62.87,36.2 62.87,34.92 66.04,34.92 66.04,37.97
MOTO3A  (via drill 0.3 pad 0.64)
  Top 0.305: R13.1 v56.9,24.13 R14.1 | v59.69,17.14 58.93,17.14
  Bottom 0.305: v59.69,17.14 59.69,21.34 v56.9,24.13
  pour Top (isolate 0.254, no thermals): 58.42,16.64 66.04,16.64 66.04,19.68 63.5,19.68 63.5,18.41 60.33,18.41 59.56,17.65 58.42,17.65
MOTO3B
  Top 0.305: D3.- D4.+ 58.55,21.34 58.55,20.83
  pour Top (isolate 0.254, rank 2, no thermals): 58.42,19.3 58.42,20.95 60.96,20.95 60.96,23.5 66.04,23.5 66.04,20.32 62.87,20.32 62.87,19.3
MOTO4A
  Top 0.305: R11.1 R12.1 58.55,8 59.82,8 60.33,8.51 60.33,11.56 60.33,11.81 | 60.33,11.81 60.33,12.7 | 60.33,11.81 59.82,12.32 | 60.33,11.81 60.71,12.19
  pour Top (isolate 0.254, rank 3, no thermals): 58.42,13.72 58.42,12.06 63.5,12.06 63.5,10.16 66.04,10.16 66.04,13.72
MOTO4B  (via drill 0.3 pad 0.64)
  Top 0.305: D1.- v56.9,10.79 D2.+ | U2.6 59.38,16.18 v59.69,15.88
  Bottom 0.305: v59.69,15.88 59.69,12.06 58.42,10.79 v56.9,10.79
  pour Top (isolate 0.254, rank 2, no thermals): 58.42,16.38 66.04,16.38 66.04,13.97 60.33,13.97 60.33,15.24 58.42,15.24
N$1
  Top 0.305: R6.2 R4.2 R5.1 C10.2
N$2
  Top 0.305: R13.2 D3.+
N$3
  Top 0.305: R14.2 D4.-
N$4
  Top 0.305: C3.2 49.02,15.62 | 49.02,15.62 C30.2 FB6.2 | U2.20 49.11,15.54 49.02,15.62
N$5  (via drill 0.3 pad 0.64)
  Top 0.406: R1.1 v27.3,15.62 | v29.84,13.78 29.84,13.26 U4.5
  Bottom 0.406: v29.84,13.78 29.84,14.86 29.08,15.62 v27.3,15.62
N$6
  Top 0.406: R1.2 C7.2
N$7  (via drill 0.3 pad 0.64)
  Top 0.406: U4.3 33.53,12.58 v33.66,12.7
  Top 0.813: C7.1 v27.13,17.21 L2.1 | v33.66,13.59 v33.66,12.7
  Bottom 0.813: v27.13,17.21 v27.83,17.21 32.32,17.21 33.66,15.88 v33.66,12.7
N$8
  Top 0.305: J1.1 64.77,24.26
  pour Top (isolate 0.254, no thermals): 61.59,24.13 66.04,24.13 66.04,26.67 63.5,26.67 63.5,27.94 59.05,27.94 59.05,25.4 61.59,25.4
N$9
  Top 0.305: U4.8 27.47,11.28 R4.1
N$10
  Top 0.305: R7.1 Q1.1
N$11
  Top 0.305: R15.2 D5.+
N$12
  Top 0.305: C9.1 32.41,9.53
  Top 0.406: U4.1 32.41,9.53 32.41,9.43
N$13
  Top 0.406: U4.7 28.33,11.93 C8.1
N$16  (via drill 0.3 pad 0.64)
  Top 0.406: R3.1 v36.26,9.53 R2.1 | 28.64,12.64 v28.57,12.7 28.7,12.58 U4.6
  Bottom 0.406: v36.26,9.53 29.84,9.53 28.57,10.79 v28.57,12.7
N$18  (via drill 0.89 pad 1.65)
  other vias: 11.43,14.61
N$19
  Top 0.305: R11.2 D1.+
N$20  (via drill 0.89 pad 1.65)
  other vias: 8.89,14.61
N$21  (via drill 0.89 pad 1.65)
  other vias: 6.35,14.61
N$22  (via drill 0.89 pad 1.65)
  other vias: 11.43,17.14
N$23
  Top 0.305: R12.2 D2.-
N$24  (via drill 0.3)
  Top 0.305: 39.08,38.44 D10.- 39.27,38.44 v39.88,39.05
  Bottom 0.305: J5.2 39.88,44.96 v39.88,39.05
N$25
  Top 0.305: R8.2 R9.2 C16.2 31.11,44.9 X1.1
N$26
  Top 0.305: R16.2 D6.-
N$27
  Top 0.305: R21.2 34.29,42.35 R9.1 C15.2 35.81,44.9 X1.2
N$28
  Top 0.305: U3.60 40.36,32.23 R10.1
N$29
  Top 0.305: R17.2 D7.+
N$30
  Top 0.305: R18.2 D8.-
N$31
  Top 0.305: U1.20 48.94,37.12 48.9,37.08 48.96,37.08 C27.2 C29.2 FB5.2
N$32  (via drill 0.3 pad 0.64)
  Top 0.305: U1.14 51.05,41.02 | U1.13 51.2,41.67 | v50.8,41.34 v50.04,41.34
  Top 0.813: F1.2 49.02,33.91 v49.28,33.66 v50.16,33.66
  Bottom 1.524: v49.28,33.66 51.31,33.66 52.23,34.58 52.23,40.43 51.32,41.34 v50.04,41.34 v50.8,41.34
  pour Top (isolate 0.254, no thermals): 49.78,41.91 52.2,41.91 52.2,40.89 49.78,40.89
  pour Top (isolate 0.254, rank 2, no thermals): 49.53,34.67 52.07,34.67 52.07,29.97 48.26,29.97 48.26,35.94 49.53,35.94
N$33  (via drill 0.89 pad 1.65)
  other vias: 8.89,17.14
N$34  (via drill 0.3 pad 0.64)
  Bottom 1.524: v49.91,12.19 51.69,12.19 53.47,13.97 53.47,21.46 51.94,22.99 v51.94,23.75
  other vias: 50.8,12.19 51.94,22.86
  pour Top (isolate 0.254, rank 2, no thermals): 48.64,11.43 52.07,11.43 52.07,13.08 48.64,13.08
  pour Top (isolate 0.254, no thermals): 50.16,19.3 52.2,19.3 52.2,24.89 50.16,24.89
N$35  (via drill 0.89 pad 1.65)
  other vias: 6.35,17.14
N$36  (via drill 0.89 pad 1.65)
  other vias: 6.35,19.68
N$37  (via drill 0.89 pad 1.65)
  other vias: 8.89,19.68
N$38  (via drill 0.89 pad 1.65)
  other vias: 11.43,19.68
N$39  (via drill 0.89 pad 1.65)
  other vias: 11.43,22.23
N$40  (via drill 0.89 pad 1.65)
  other vias: 8.89,22.23
N$41  (via drill 0.89 pad 1.65)
  other vias: 6.35,22.23
N$42  (via drill 0.89 pad 1.65)
  other vias: 11.43,24.77
N$43  (via drill 0.89 pad 1.65)
  other vias: 8.89,24.77
N$44
  Top 0.305: R23.2 PWR.-
N$45  (via drill 0.89 pad 1.65)
  other vias: 6.35,24.77
N$46  (via drill 0.89 pad 1.65)
  other vias: 6.35,27.3
N$47  (via drill 0.89 pad 1.65)
  other vias: 8.89,27.3
N$48  (via drill 0.89 pad 1.65)
  other vias: 11.43,27.3
N$49  (via drill 0.89 pad 1.65)
  other vias: 6.35,29.84
N$50  (via drill 0.89 pad 1.65)
  other vias: 8.89,29.84
N$51  (via drill 0.89 pad 1.65)
  other vias: 11.43,29.84
N$52  (via drill 0.89 pad 1.65)
  other vias: 6.35,32.38
N$53  (via drill 0.89 pad 1.65)
  other vias: 6.35,34.92
N$54  (via drill 0.89 pad 1.65)
  other vias: 6.35,37.47
N$55  (via drill 0.89 pad 1.65)
  other vias: 6.35,40.01
N$56  (via drill 0.89 pad 1.65)
  other vias: 6.35,42.55
N$57  (via drill 0.89 pad 1.65)
  other vias: 8.89,42.55
N$58  (via drill 0.89 pad 1.65)
  other vias: 11.43,42.55
N$59  (via drill 0.89 pad 1.65)
  other vias: 13.97,42.55
N$60  (via drill 0.3)
  Top 0.305: v37.85,37.47 D9.-
  Bottom 0.305: J8.23 32.38,3.17 32.38,5.08 33.53,6.22 43.56,6.22 45.09,7.75 45.09,18.92 43.05,20.95 35.94,20.95 30.48,26.42 30.48,34.42 33.53,37.47 v37.85,37.47
N$61  (via drill 0.89 pad 1.65)
  other vias: 8.89,40.01
N$62  (via drill 0.89 pad 1.65)
  other vias: 11.43,40.01
N$63  (via drill 0.89 pad 1.65)
  other vias: 13.97,40.01
N$65  (via drill 0.89 pad 1.65)
  other vias: 8.89,37.47
N$66  (via drill 0.89 pad 1.65)
  other vias: 11.43,37.47
N$67  (via drill 0.89 pad 1.65)
  other vias: 13.97,37.47
N$69  (via drill 0.89 pad 1.65)
  other vias: 8.89,34.92
N$70  (via drill 0.89 pad 1.65)
  other vias: 8.89,32.38
N$71  (via drill 0.89 pad 1.65)
  other vias: 11.43,34.92
N$72  (via drill 0.89 pad 1.65)
  other vias: 11.43,32.38
N$73  (via drill 0.89 pad 1.65)
  other vias: 13.97,34.92
N$74  (via drill 0.89 pad 1.65)
  other vias: 13.97,32.38
N$77  (via drill 0.89 pad 1.65)
  other vias: 13.97,29.84
NRST  (via drill 0.3, 0.3 pad 0.64)
  Top 0.305: U3.7 31.86,37.35 v31.11,38.1 C24.2 | D9.+ 38.35,40.04 | 38.35,40.04 D10.+ 40.69,40.04 K1.2 K1.1 | v38.42,40.51 38.42,40.11 38.35,40.04
  Bottom 0.305: v31.11,38.1 32.13,39.12 37.02,39.12 v38.42,40.51
OSC_IN
  Top 0.305: U3.5 32.87,37.82 R21.1
OSC_OUT
  Top 0.305: U3.6 32.37,38.91 R8.1
PA0  (via drill 0.3 pad 0.64)
  Top 0.305: U3.14 28.36,34.5 28.96,33.91 v31.11,33.91 | U2.17 50.63,17.48 v50.16,17.02
  Bottom 0.305: v31.11,33.91 31.11,26.67 36.2,21.59 46.86,21.59 48.9,19.56 48.9,18.16 50.04,17.02 v50.16,17.02
PA1
  Top 0.305: U3.15 27.86,37.54 27.3,38.1 25.91,38.1 R19.1
  Top 0.406: R20.1 C32.2 R19.1
PA2  (via drill 0.3 pad 0.64)
  Top 0.305: U3.16 27.3,37.27 27.11,37.47 v24.77,37.47
  Bottom 0.305: v24.77,37.47 24.51,37.21 24.51,27.18 21.46,24.13 J10.5
PA3  (via drill 0.3 pad 0.64)
  Top 0.305: U3.17 23.5,34.29 v22.86,34.92
  Bottom 0.305: v22.86,34.92 22.86,28.45 21.08,26.67 J10.6
PA4
  Top 0.305: U3.20 24.17,32.73 21.97,34.92 21.97,40.26 J12.1
PA5
  Top 0.305: U3.21 23.9,32.23 21.46,34.67 21.46,38.23 J12.2
PA6
  Top 0.305: U3.22 23.64,31.73 20.95,34.42 20.95,36.2 J12.3
PA7
  Top 0.305: U3.23 23.38,31.23 J12.4
PA8  (via drill 0.3 pad 0.64)
  Top 0.305: U3.41 31.36,25.66 30.99,26.04 27.18,26.04 26.16,25.02 v24.77,25.02
  Bottom 0.305: v24.77,25.02 21.46,21.72 21.46,18.29 J10.2
PA9  (via drill 0.3 pad 0.64)
  Top 0.305: U3.42 31.86,23.55 v31.69,23.37
  Bottom 0.305: J8.22 28.57,5.08 30.73,7.24 42.8,7.24 43.81,8.26 43.81,18.41 42.55,19.68 35.21,19.68 31.69,23.21 v31.69,23.37
PA10  (via drill 0.3 pad 0.64)
  Top 0.305: U3.43 32.37,23.52 v32.51,23.37
  Bottom 0.305: J8.21 29.84,3.17 29.84,5.08 31.5,6.73 43.24,6.73 44.45,7.94 44.45,18.67 42.8,20.32 35.56,20.32 v32.51,23.37
PA11  (via drill 0.3 pad 0.64)
  Top 0.305: U3.44 32.87,26.06 32.26,26.67 26.92,26.67 25.91,25.65 v25.4,25.65
  Bottom 0.305: v25.4,25.65 25.4,24.77 21.97,21.34 21.97,16.26 J10.1
PA12  (via drill 0.3 pad 0.64)
  Top 0.305: U3.45 33.37,28.92 v33.66,29.21 | v48.51,44.07 52.83,44.07 53.98,42.93 53.98,40.13 52.92,39.08 U1.17
  Bottom 0.305: v48.51,44.07 48.26,43.81 46.48,43.81 43.81,41.15 43.81,30.97 40.15,27.3 34.54,27.3 33.66,28.19 v33.66,29.21
PA13  (via drill 0.3 pad 0.64)
  Top 0.305: U3.46 33.87,28.15 v34.92,29.21
  Bottom 0.305: J5.4 41.91,41.91 41.91,31.88 39.24,29.21 v34.92,29.21
PA14  (via drill 0.3 pad 0.64)
  Top 0.305: U3.49 35.56,26.67 34.92,27.3 v34.92,27.94
  Bottom 0.305: J5.6 50.16,45.09 48.51,45.09 47.88,44.45 46.23,44.45 43.18,41.4 43.18,31.3 39.83,27.94 v34.92,27.94
PA15  (via drill 0.3 pad 0.64)
  Top 0.305: U3.50 36.02,27.23 35.56,27.69 v35.56,28.57
  Bottom 0.305: v35.56,28.57 39.53,28.57 42.55,31.59 42.55,41.66 45.97,45.09 47.62,45.09 J5.5
PB0  (via drill 0.3 pad 0.64)
  Top 0.305: U3.26 31.64,29.73 v31.75,29.84 | U2.23 v50.17,13.59 v50.16,13.59
  Bottom 0.305: v31.75,29.84 32.64,29.84 33.02,29.46 33.02,27.43 35.69,24.77 48.13,24.77 52.07,20.83 52.07,14.61 51.05,13.59 v50.16,13.59
PB1  (via drill 0.3 pad 0.64)
  Top 0.305: U2.15 50.22,18.79 v50.16,18.73 | v32.38,29.21 25.23,29.21 U3.27
  Bottom 0.305: v32.38,29.21 32.38,27.18 36.7,22.86 47.37,22.86 50.16,20.07 v50.16,18.73
PB2  (via drill 0.3 pad 0.64)
  Top 0.305: U3.28 31.59,28.73 v31.75,28.57 | U2.16 50.39,18.14 v50.16,17.91
  Bottom 0.305: v31.75,28.57 31.75,26.92 36.45,22.23 47.12,22.23 49.53,19.81 49.53,18.41 50.04,17.91 v50.16,17.91
PB3  (via drill 0.3 pad 0.64)
  Top 0.305: v42.42,43.43 52.58,43.43 53.34,42.67 53.34,40.39 52.68,39.73 U1.16 | U3.55 35.67,29.73 v35.56,29.84
  Bottom 0.305: v35.56,29.84 38.91,29.84 41.27,32.21 41.27,42.29 v42.42,43.43
PB4  (via drill 0.3 pad 0.64)
  Top 0.305: U3.56 37.97,30.23 38.73,29.46 v38.73,26.67 | v50.8,35.18 U1.23
  Bottom 0.305: v38.73,26.67 40.43,26.67 44.45,30.69 44.45,35.71 46.08,37.34 50.16,37.34 50.8,36.7 v50.8,35.18
PB5  (via drill 0.3 pad 0.64)
  Top 0.305: U3.57 35.17,30.73 v34.92,30.48 | U1.15 52.44,40.38 52.7,40.64 52.7,42.42 52.32,42.8 v40.64,42.8
  Bottom 0.305: v34.92,30.48 38.7,30.48 40.64,32.42 v40.64,42.8
PB6  (via drill 0.3 pad 0.64)
  Top 0.305: U3.58 37.98,31.23 39.37,29.84 v39.37,19.05 | J8.19 24.77,3.17 24.77,5.21 24.32,5.65 R24.2
  Bottom 0.305: J8.19 27.3,3.17 27.3,5.08 29.97,7.75 39.81,7.75 41.27,9.21 41.27,18.41 40.64,19.05 v39.37,19.05
PB7  (via drill 0.3, 0.3 pad 0.64)
  Top 0.305: U3.59 38.37,31.73 40.01,30.1 v40.01,18.41 | v28.57,7.62 28.07,8.13 R22.2
  Bottom 0.305: J8.20 26.04,5.08 v28.57,7.62 29.21,8.26 39.37,8.26 40.64,9.53 40.64,17.78 v40.01,18.41
PB8  (via drill 0.3 pad 0.64)
  Top 0.305: U3.61 27.65,32.73 v27.3,32.38
  Bottom 0.305: v27.3,32.38 25.78,30.86 25.78,26.92 20.95,22.1 20.95,20.32 J10.3
PB9  (via drill 0.3 pad 0.64)
  Top 0.305: U3.62 26.88,33.23 v26.67,33.02
  Bottom 0.305: v26.67,33.02 25.15,31.5 25.15,27.05 J10.4
PB10
  Top 0.305: U3.29 22.06,28.23 20.95,29.34 20.95,31.11 J12.5
PB11
  Top 0.305: U3.30 21.8,27.73 J12.6
PB12  (via drill 0.3 pad 0.64)
  Top 0.305: U3.33 27.3,22.61 29.08,20.83 35.76,20.83 38.1,23.17 v38.1,24.13 | U2.22 50.81,14.23 v50.8,14.22
  Bottom 0.305: v50.8,14.22 51.44,14.86 51.44,20.57 47.88,24.13 v38.1,24.13
PB13  (via drill 0.3 pad 0.64)
  Top 0.305: U3.34 27.86,22.81 29.21,21.46 35.43,21.46 v37.47,23.5 | U2.21 50.19,14.88 v50.16,14.86
  Bottom 0.305: v50.16,14.86 50.8,15.49 50.8,20.32 47.62,23.5 v37.47,23.5
PB14  (via drill 0.3 pad 0.64)
  Top 0.305: U3.35 28.36,23.07 29.34,22.1 35.12,22.1 36.2,23.18 v36.2,25.4 | U1.22 50.3,35.83 v50.04,35.56
  Bottom 0.305: v36.2,25.4 40.99,25.4 45.72,30.13 45.72,35.09 46.57,35.94 49.66,35.94 v50.04,35.56
PB15  (via drill 0.3 pad 0.64)
  Top 0.305: U3.36 28.86,23.33 29.46,22.73 34.82,22.73 35.56,23.47 v35.56,26.04 | U1.21 50.19,36.48 v50.16,36.45
  Bottom 0.305: v35.56,26.04 40.7,26.04 45.09,30.42 45.09,35.42 46.11,36.45 v50.16,36.45
STBY  (via drill 0.3 pad 0.64)
  Top 0.305: U1.19 50.49,37.77 v50.16,38.1 | v44.45,20.95 43.18,20.95 42.55,21.59 42.55,35.43 43.18,36.07 44.83,36.07 45.59,36.83 v45.59,38.1 | v50.16,16.19 50.17,16.18 U2.19 52.4,16.18 52.83,15.75 52.83,11.18 52.45,10.79 45.97,10.79 45.09,11.68 SW1.COM
  Bottom 0.305: v50.16,38.1 v45.59,38.1 | v50.16,16.19 49.97,16.19 48.26,17.91 48.26,19.3 46.61,20.95 v44.45,20.95
VBAT  (via drill 0.3 pad 0.64)
  Top 0.305: 35.12,11.87 35.12,11.75 C5.2
  Top 0.406: U4.2 33.41,11.93 | 33.41,11.93 35.06,11.93 35.12,11.87 | 33.41,11.93 33.78,11.56 | F1.1 v47.5,34.67 | R7.2 v54.48,28.96
  Top 0.61: R19.2 v24.07,41.47 | v38.73,41.91 39.62,41.02 45.34,41.02 46.48,39.88 46.48,34.92 v46.74,34.67 | F1.1 47.24,35.56
  Top 0.813: F2.1 42.67,12.7 41.59,11.62 C6.2 C5.2 34.04,11.62 33.97,11.68 33.97,10.9 | R2.2 33.97,10.9 | 33.97,10.9 34.01,10.9 34.8,11.68
  Bottom 0.305: 48.01,11.81 v47.88,11.81 | 47.88,11.68 v47.88,11.81 | 47.75,11.56 47.75,11.68 v47.88,11.81 | v47.88,11.81 v47.24,11.81
  Bottom 0.406: v47.5,34.67 47.12,34.67 v46.74,34.67
  Bottom 0.61: v24.07,41.47 25.02,42.42 38.23,42.42 v38.73,41.91 | 55.5,29.72 55.63,29.84
  Bottom 1.524: 55.63,29.84 53.59,29.84 | 53.59,29.84 48.9,29.84 47.12,31.62 47.12,34.67 | 53.59,29.84 54.74,28.7 | 55.63,26.42 55.63,13.08 52.7,10.16 49.15,10.16 47.75,11.56
  pour Bottom (isolate 0.254, no thermals): 53.98,30.48 66.04,30.48 66.04,27.94 56.52,27.94 56.52,25.4 53.98,25.4
  pour Top (isolate 0.254, no thermals): 46.29,36.07 47.88,36.07 47.88,34.29 46.29,34.29
  pour Top (isolate 0.254, no thermals): 46.35,11.43 48.26,11.43 48.26,13.08 46.35,13.08
VDD  (via drill 0.3 pad 0.64)
  Top 0.406: U3.32 24.32,26.67 C19.2 | U3.1 34.92,38.29 C22.2 36.39,39.75 v36.7,39.75 36.96,39.5 36.96,37.08 39.12,34.92 C21.2 U3.64
  Top 0.61: FB3.1 v26.35,41.61 26.35,42.23 26.29,42.29 26.29,42.35 FB2.2 C20.2 | C19.2 23.11,25.53 v22.23,26.42
  Bottom 0.61: v22.23,26.42 23.75,27.94 23.75,39.88 25.48,41.61 v26.35,41.61 34.46,41.61 36.32,39.75 v36.7,39.75
VDD_3V3B
  Top 0.61: J8.3 J8.4 5.71,7.49 C13.2 C33.2 FB4.2
VDD_5V
  Top 0.813: J8.5 J8.6 8.26,5.08 9.53,6.35 14.35,6.35 16.13,8.13 | FB1.2 C31.2 16.13,8.13 | 16.13,8.13 C2.2
VDDA
  Top 0.305: FB3.2 C18.2 C17.2 29.53,38.16 28.86,37.5 U3.13

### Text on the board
tPlace: 2 | 1 | 40 | 20 | 20 | 40 | 2 | 1
bPlace: BAT+ | Maximum input / voltage:DC15V | Motor Bridge Cape | BAT- | v1.0 07/17/2015 | by Seeed Studio | www.seeedstudio.com
tNames: 3V3 | GND | NC | RX2 | CLK / TX2 | PA4 | NRST | SWDIO | A5 | Motor1 | A6 | RST | GND | A7 | Motor2 | B10 | B11 | + | A3 | A2 | B9 | B8 | SERVO | Motor3 | WORKING | A8 | A11 | Motor4 | PWR | 5V | IO | GND | STBY

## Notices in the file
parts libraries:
moudle-new: This work is licensed under the Creative Commons Attribution 4.0 International License.
To view a copy of this license,visit:
http://creativecommons.org/licenses/by-sa/4.0
moudle-new: CC-BY-SA
